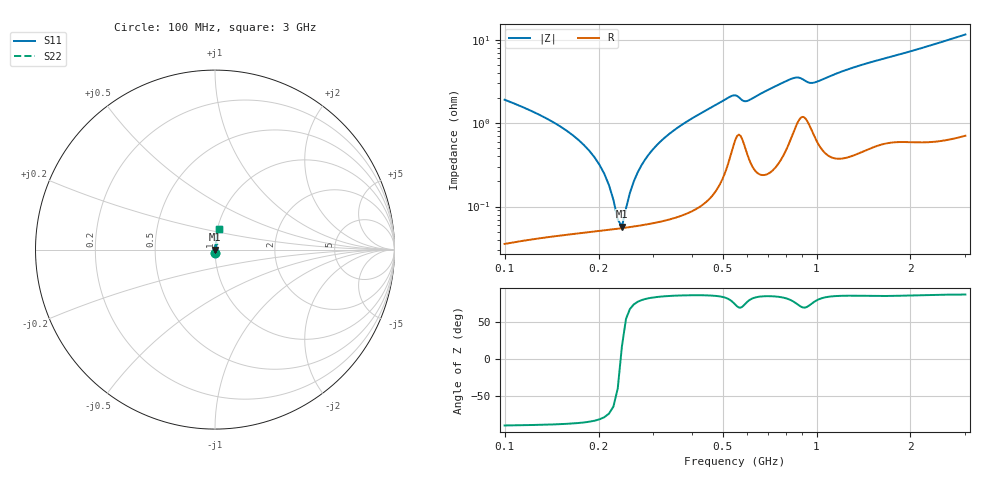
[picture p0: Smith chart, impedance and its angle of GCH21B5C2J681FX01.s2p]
!Murata Part Number: GCH21B5C2J681FX01
!These Parameters are Measured in Series Mode Connection
!Data Generated on Jun 19, 2026
!  o--ll--o
!Port1  Port2
!  o------o
!Operation Temp=25[degC], DC Bias Voltage=0[V]
!Freq. Start=100[MHz] Stop=3[GHz] 401[Steps]
# Hz S RI R 50
!Freq.(Hz) S11(Real) S11(Imag) S21(Real) S21(Imag) S12(Real) S12(Imag) S22(Real) S22(Imag)
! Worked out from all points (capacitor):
!   401 points, 100 MHz to 3 GHz, reference 50 ohm
!   read as one part in series: C = 685 pF near 114.5 MHz
!   lowest |Z| = 57.7 mohm at 237.8 MHz (marker M1)
!   series resonance near 235.7 MHz, so ESL is about 670 pH
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1e8  0.00072 -0.019  0.9993 0.019  0.9993 0.019  0.00072 -0.019
1.435e8  0.000543 -0.0102  0.9995 0.0102  0.9995 0.0102  0.000543 -0.0102
1.7975e8  0.000515 -0.00542  0.9995 0.00542  0.9995 0.00542  0.000515 -0.00542
2.015e8  0.00052 -0.00312  0.9995 0.00312  0.9995 0.00312  0.00052 -0.00312
2.2325e8  0.000536 -0.00108  0.9995 0.00108  0.9995 0.00108  0.000536 -0.00108
2.3775e8  0.000551 0.00017  0.9994 -0.00017  0.9994 -0.00017  0.000551 0.00017
2.45e8  0.00056 0.000768  0.9994 -0.000768  0.9994 -0.000768  0.00056 0.000768
2.6675e8  0.000592 0.00247  0.9994 -0.00247  0.9994 -0.00247  0.000592 0.00247
2.8125e8  0.000618 0.00355  0.9994 -0.00355  0.9994 -0.00355  0.000618 0.00355
3.03e8  0.000663 0.00509  0.9993 -0.00509  0.9993 -0.00509  0.000663 0.00509
3.3925e8  0.00076 0.00752  0.9992 -0.00752  0.9992 -0.00752  0.00076 0.00752
4.045e8  0.00104 0.0117  0.999 -0.0117  0.999 -0.0117  0.00104 0.0117
5.205e8  0.00363 0.0197  0.9964 -0.0197  0.9964 -0.0197  0.00363 0.0197
5.495e8  0.00673 0.0203  0.9933 -0.0203  0.9933 -0.0203  0.00673 0.0203
5.8575e8  0.00582 0.0173  0.9942 -0.0173  0.9942 -0.0173  0.00582 0.0173
8.395e8  0.00848 0.0331  0.9915 -0.0331  0.9915 -0.0331  0.00848 0.0331
9.6275e8  0.00908 0.0286  0.9909 -0.0286  0.9909 -0.0286  0.00908 0.0286
1.0715e9  0.00545 0.0343  0.9946 -0.0343  0.9946 -0.0343  0.00545 0.0343
1.55e9  0.00829 0.0549  0.9917 -0.0549  0.9917 -0.0549  0.00829 0.0549
2.03575e9  0.0112 0.0724  0.9888 -0.0724  0.9888 -0.0724  0.0112 0.0724
2.5215e9  0.0147 0.0919  0.9853 -0.0919  0.9853 -0.0919  0.0147 0.0919
3e9  0.0198 0.1122  0.9802 -0.1122  0.9802 -0.1122  0.0198 0.1122
